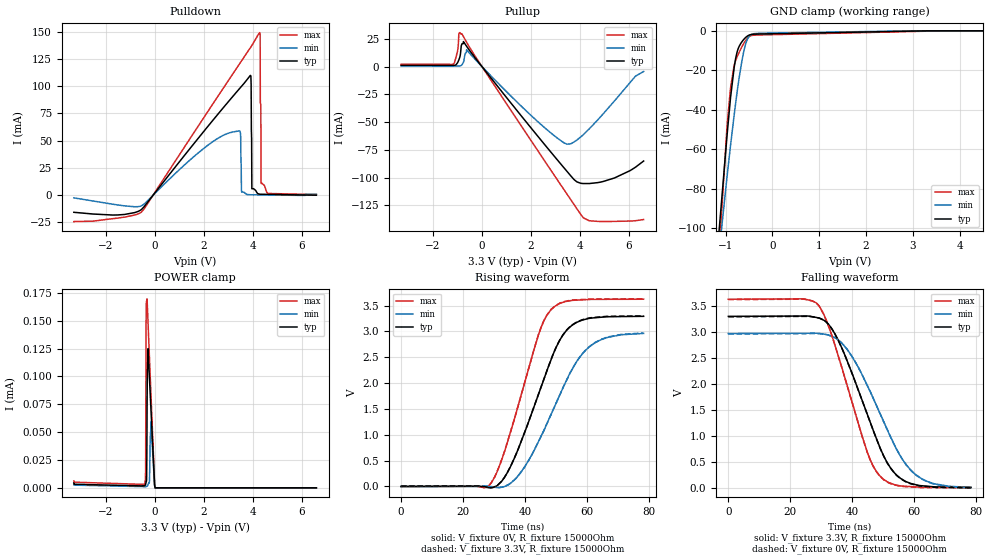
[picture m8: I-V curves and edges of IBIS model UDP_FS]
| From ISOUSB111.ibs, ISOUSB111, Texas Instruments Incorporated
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[Model]   UDP_FS
Model_type   I/O
Polarity   Non-Inverting
Enable   Active-Low
Vinl = 0.8
Vinh = 2
Vmeas = 1.65
Vref = 1.65
Cref = 7pF
Rref = 15000
|   typ   min   max
C_comp   8pF   5pF   10pF
[Voltage Range]   3.3   2.97   3.63
[Temperature Range]   27   150   -40
[Pullup Reference]   3.3   2.97   3.63
[Pulldown Reference]   -0   0   0
[Power Clamp Reference]   3.3   2.97   3.63
[GND Clamp Reference]   0   0   0
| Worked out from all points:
|   slope of the pulldown table from 0 to 0.495 V, typ, clamps not added: 34.8 ohm
|   slope of the pullup table from 0 to 0.495 V, typ, clamps not added: 35.9 ohm
|   falling waveform, V_fixture 3.3V, R_fixture 15000Ohm: 20-80 % time 12.8ns typ, 14.3ns min, 11.1ns max; typ from 3.3 V to 0.007 V
|   rising waveform, V_fixture 0V, R_fixture 15000Ohm: 20-80 % time 12.3ns typ, 14.2ns min, 10.5ns max; typ from 0 V to 3.29 V
|   rising waveform, V_fixture 3.3V, R_fixture 15000Ohm: 20-80 % time 12.3ns typ, 14.2ns min, 10.5ns max; typ from 0.007 V to 3.3 V
|   falling waveform, V_fixture 0V, R_fixture 15000Ohm: 20-80 % time 12.8ns typ, 14.3ns min, 11ns max; typ from 3.29 V to 0 V
[Pulldown]
|   Voltage   I(typ)   I(min)   I(max)
-3.3V     -16.09mA   -2.786mA   -24.62mA
-537.9mV  -13.47mA   -10.11mA   -15.82mA
3.452V    97.48mA    58.87mA    120.2mA
3.551V    100.1mA    2.363mA    123.5mA
3.907V    109.9mA    72.16uA    135.5mA
3.937V    101.8mA    61.77uA    136.5mA
3.967V    5.59mA     51.41uA    137.5mA
4.283V    617.9uA    -57.09uA   149.4mA
4.303V    541.1uA    -63.73uA   147.9mA
4.313V    537.2uA    -67.05uA   84.09mA
4.353V    520.1uA    -80.27uA   10.29mA
6.6V      -360.3uA   452.3uA    310.5uA
[GND Clamp]
|   Voltage   I(typ)   I(min)   I(max)
-3.3V     -1.288A    -1.122A    -1.582A
-1.3V     -147.2mA   -148.5mA   -173mA
-973.5mV  -54.42mA   -74.96mA   -50.1mA
-894.3mV  -33.89mA   -58.12mA   -28.9mA
-815.1mV  -18.32mA   -42.37mA   -17.26mA
-785.4mV  -14.06mA   -36.76mA   -15.01mA
-735.9mV  -9.386mA   -27.92mA   -12.19mA
-627mV    -4.803mA   -12.27mA   -7.026mA
-567.6mV  -3.283mA   -6.365mA   -4.738mA
-498.3mV  -2.184mA   -2.858mA   -2.959mA
-240.9mV  -1.597mA   -1.202mA   -2.074mA
6.6V      0A         0A         0A
[Pullup]
|   Voltage   I(typ)   I(min)   I(max)
-3.3V     1.143mA    463.2uA    2.099mA
-1.181V   1.062mA    442.5uA    1.998mA
-993.3mV  3.495mA    442.2uA    14.21mA
-933.9mV  6.482mA    535.8uA    30.27mA
-815.1mV  20.52mA    1.636mA    29.45mA
-627mV    18.33mA    15.2mA     21.98mA
1.957V    -53.99mA   -43.05mA   -65.07mA
3.491V    -94.94mA   -69.92mA   -115.6mA
3.868V    -103.7mA   -66.32mA   -127.8mA
4.382V    -105.4mA   -56.09mA   -138.9mA
5.412V    -100.3mA   -30.9mA    -139.5mA
6.6V      -85.09mA   -4.411mA   -137.8mA
[POWER Clamp]
|   Voltage   I(typ)   I(min)   I(max)
-3.3V     4.356uA    3.599uA    6.246uA
-409.2mV  1.975uA    1.064uA    3.581uA
-369.6mV  3.167uA    1.032uA    15.05uA
-349.8mV  5.429uA    1.011uA    150.3uA
-330mV    6.968uA    1.294uA    167.9uA
-310.2mV  73.23uA    1.416uA    169.7uA
-300.3mV  102.4uA    1.539uA    164.2uA
-270.6mV  124.9uA    2.826uA    148uA
-211.2mV  97.43uA    7.019uA    115.9uA
-151.8mV  70.29uA    59.27uA    83.87uA
16.5mV    0A         0A         0A
6.6V      0A         0A         0A
[Ramp]
R_load = 15000
|   typ   min   max
dV/dt_r   1.97481/1.22575e-08   1.77642/1.41863e-08   2.17309/1.05057e-08
dV/dt_f   1.97495/1.27511e-08   1.77633/1.42545e-08   2.17324/1.10345e-08
[Falling Waveform]
V_fixture = 3.3V
V_fixture_min = 2.97V
V_fixture_max = 3.63V
R_fixture = 15000Ohm
C_fixture = 0F
|   Time   V(typ)   V(min)   V(max)
0s        3.299V     2.969V     3.629V
28.25ns   3.28V      2.975V     3.563V
33.36ns   3.065V     2.916V     2.942V
38.41ns   2.437V     2.661V     1.961V
44.89ns   1.414V     1.968V     684.3mV
48.66ns   821.2mV    1.475V     247.8mV
53.93ns   270mV      788.7mV    57.41mV
60.63ns   58.78mV    248.8mV    17.93mV
66.4ns    20.14mV    80mV       10.02mV
78.33ns   7.45mV     8.552mV    6.827mV
[Rising Waveform]
V_fixture = 0V
V_fixture_min = 0V
V_fixture_max = 0V
R_fixture = 15000Ohm
C_fixture = 0F
|   Time   V(typ)   V(min)   V(max)
0s        -34.84uV   -43.96uV   -29.01uV
28.25ns   -23.55mV   -2.757mV   10.06mV
31.69ns   54.41mV    -23.07mV   386.4mV
35.38ns   390.3mV    63.84mV    1.061V
44.36ns   1.781V     869mV      2.933V
48.16ns   2.409V     1.358V     3.4V
53.3ns    3.009V     2.038V     3.579V
60.16ns   3.243V     2.667V     3.615V
66.92ns   3.283V     2.887V     3.62V
78.33ns   3.291V     2.961V     3.622V
[Rising Waveform]
V_fixture = 3.3V
V_fixture_min = 2.97V
V_fixture_max = 3.63V
R_fixture = 15000Ohm
C_fixture = 0F
|   Time   V(typ)   V(min)   V(max)
0s        7.45mV     8.552mV    6.827mV
28.25ns   -16.15mV   5.411mV    12.5mV
31.69ns   55.57mV    -18.12mV   389mV
35.38ns   391.6mV    65.07mV    1.064V
44.36ns   1.783V     866.9mV    2.937V
48.16ns   2.412V     1.356V     3.405V
53.3ns    3.014V     2.037V     3.585V
60.16ns   3.25V      2.671V     3.622V
66.92ns   3.291V     2.894V     3.627V
78.33ns   3.299V     2.969V     3.629V
[Falling Waveform]
|Gnd
V_fixture = 0V
V_fixture_min = 0V
V_fixture_max = 0V
R_fixture = 15000Ohm
C_fixture = 0F
|   Time   V(typ)   V(min)   V(max)
0s        3.291V     2.961V     3.622V
28.25ns   3.278V     2.968V     3.564V
33.36ns   3.066V     2.916V     2.94V
38.41ns   2.436V     2.663V     1.958V
44.89ns   1.41V      1.968V     680.6mV
48.66ns   817.9mV    1.474V     242.8mV
53.93ns   264.9mV    786.1mV    51.24mV
60.63ns   52.08mV    243.2mV    11.09mV
66.4ns    12.9mV     72.68mV    3.213mV
78.33ns   -34.84uV   -43.96uV   -29.01uV
